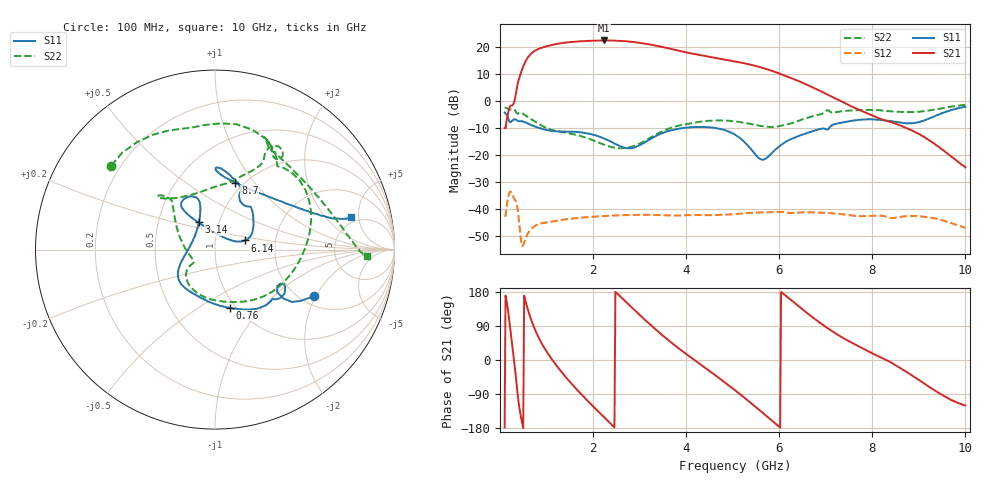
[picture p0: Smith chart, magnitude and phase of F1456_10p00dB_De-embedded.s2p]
! Integrated Device Technology
! Corporate Headquarters
! 6024 Silver Creek Valley Road
! San Jose, CA 95138  USA
! Phone:  1-408-284-8200
! Toll Free:  1-800-223-1366
! Webpage:  http://www.idt.com/
! Timing and RF Division
! 515 Groton Road, Suite 102
! Westford, MA 01886-6024
! Device:  F1456
! Description: 6-bit 0.5 dB Transmit Variable Gain Amplifier
! Frequency:  2100.0 -  2950.00 MHz
! Package:  6x6 mm Thin QFN Plastic Package: 28 pin
! State:  20
! Atten State:  10.0 dB
! Voltage:  +5.00 Volts
! Current:  217.037 mA
! Data:  The device was measured on a the F1455 evaluation board which has
!  individual transmission lines to the RF pins.  Data was collected
!  using a calibrated network analyzer.  The evaluation board was
!  de-embedded using a TRL calibration technique.
!  The reference plane is the edge of the package pin.
!  Pin  1 = CSb
!  Pin  2 = DATA
!  Pin  3 = CLK
!  Pin  4 = RSET
!  Pin  5 = GND
!  Pin  6 = RFIN  = Port 1
!  Pin  7 = GND
!  Pin  8 = NC
!  Pin  9 = NC
!  Pin 10 = NC
!  Pin 11 = NC
!  Pin 12 = NC
!  Pin 13 = NC
!  Pin 14 = /STBY
!  Pin 15 = GND
!  Pin 16 = RFOUT  = Port 2
!  Pin 17 = GND
!  Pin 18 = NC
!  Pin 19 = NC
!  Pin 20 = NC
!  Pin 21 = GND
!  Pin 22 = NC
!  Pin 23 = GND
!  Pin 24 = NC
!  Pin 25 = NC
!  Pin 26 = NC
!  Pin 27 = GND
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# GHz S dB R 50
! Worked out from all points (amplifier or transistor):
!   496 points, 100 MHz to 10 GHz, reference 50 ohm
!   highest |S21| = 22.3 dB at 2.24 GHz (marker M1)
!   |S21| within 3 dB of that: 845.8 MHz to 3.645 GHz (2.799 GHz wide, 125 % of centre)
!   unconditionally stable (mu >= 1): start of sweep to end of sweep
!   at 1.74 GHz: K = 5.09, MAG = 22.5 dB, |S12| = -43.1 dB
!   at 5.06 GHz: K = 8.98, MAG = 15.6 dB, |S12| = -41.7 dB
!   at 10 GHz: K = 206.71, MAG = -15.0 dB, |S12| = -46.9 dB
!   S11 on the Smith chart (normalised r, x): 100 MHz: 2.34, -1.94; 760 MHz: 0.94, -0.68; 3.14 GHz: 0.80, +0.26; 6.14 GHz: 1.40, +0.15; 8.7 GHz: 0.92, +0.80; 10 GHz: 4.34, +4.00
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0.1  -4.29 -25.2  -9.96 -177.8  -42.36 46.2  -2.58 141.0
0.32  -6.78 -32.3  0.56 -19.9  -36.50 -138.8  -3.37 64.9
0.42  -7.48 -41.2  8.72 -128.2  -46.37 140.2  -4.35 44.7
0.58  -8.19 -58.7  15.52 141.5  -49.56 175.0  -5.79 4.2
0.76  -9.54 -75.9  18.60 78.0  -46.08 131.4  -7.68 -29.5
0.98  -10.62 -96.1  20.07 26.6  -44.88 90.5  -9.86 -65.2
1.2  -11.23 -112.8  20.97 -12.3  -44.28 65.1  -11.06 -92.8
1.5  -11.35 -130.0  21.70 -57.4  -43.49 39.1  -12.01 -121.4
1.76  -11.66 -140.9  22.03 -92.1  -43.05 21.1  -13.09 -136.8
2.24  -13.90 -159.4  22.31 -151.3  -42.48 -7.1  -16.17 -147.6
2.64  -17.10 171.3  22.10 160.9  -42.18 -28.5  -17.44 -154.3
3.14  -14.97 120.0  21.08 103.0  -42.03 -54.1  -14.47 167.0
3.4  -12.55 110.3  20.24 74.7  -42.12 -66.8  -11.98 148.3
3.72  -10.65 108.3  19.02 42.2  -42.30 -81.0  -9.65 135.1
4.08  -9.74 114.4  17.63 8.9  -42.19 -95.6  -8.35 131.8
5.06  -12.56 127.1  14.55 -80.7  -41.73 -136.8  -7.57 136.5
5.62  -21.65 69.6  12.31 -136.8  -41.13 -166.7  -9.30 120.5
6.14  -15.10 16.9  9.17 169.5  -41.11 161.2  -8.78 83.9
6.7  -11.29 38.2  5.14 114.2  -41.15 130.3  -5.74 62.7
8.36  -7.36 87.4  -7.64 -3.6  -43.13 58.0  -3.81 62.5
8.7  -8.22 73.0  -9.79 -28.7  -42.57 50.1  -4.10 51.4
10  -2.15 13.3  -24.51 -119.8  -46.86 -29.2  -1.46 -2.5
